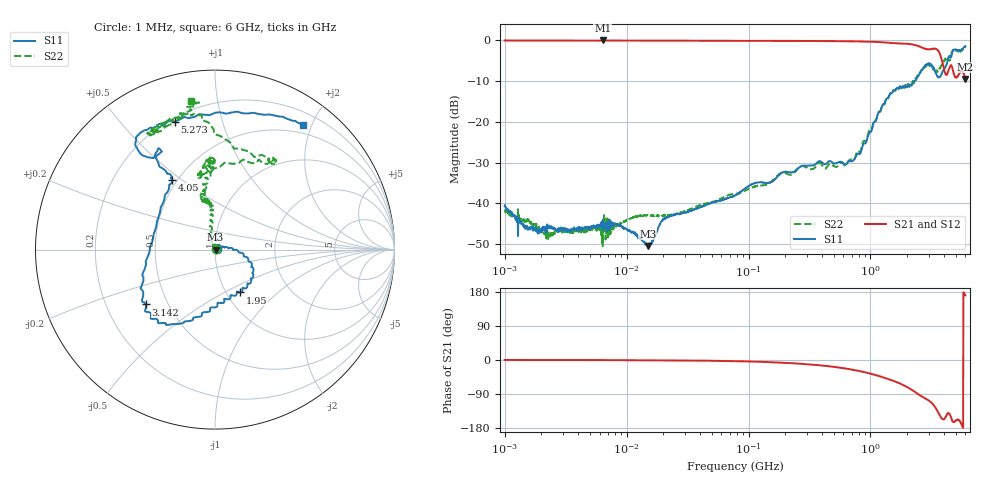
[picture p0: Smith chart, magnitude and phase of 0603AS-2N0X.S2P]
!s-Parameter Generated by FASTRON Sdn. Bhd.
!FASTRON P/N : 0603AS-2N0X
!Keysight Technologies: E5071C_MY46733604_B.14.02
!Date: Tue Nov 21 15:46:42 2023
!Version  :Rev01  Tue Nov 21 15:46:42 2023
!Data & Calibration Information:
!Freq  S11:SOLT2(ON)  S21:SOLT2(ON)  S12:SOLT2(ON)  S22:SOLT2(ON)
!PortZ  Port1:50+j0  Port2:50+j0
!When reading reference impedance value at option line is always used.
! Remarks : This data is being provided solely for informational purposes.
# Hz S dB R 50
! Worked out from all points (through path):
!   1601 points, 1 MHz to 6 GHz, reference 50 ohm
!   highest |S21| = -0.02 dB at 6.378 MHz (marker M1); lowest = -9.5 dB at 6 GHz (marker M2)
!   group delay of S21, straight-line fit = 94.1 ps
!   lowest |S11| = -50.5 dB at 14.93 MHz (marker M3), VSWR 1.01, Z = 50.3 + j7.26e-05 ohm
!   |S11| at or under -10 dB: start of sweep to 2.301 GHz
!   |S22| runs from -50.5 to -1.6 dB; largest |S21 - S12| = 0.0075
!   S11 on the Smith chart (normalised r, x): 1 MHz: 1.02, +0.01; 1.95 GHz: 1.16, -0.60; 3.142 GHz: 0.38, -0.30; 4.05 GHz: 0.47, +0.46; 5.273 GHz: 0.22, +0.71; 6 GHz: 0.37, +1.86
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1000000  -40.68 15.9  -0.04 0.1  -0.06 0.1  -41.49 20.4
1554926  -46.48 3.0  -0.04 -0.1  -0.06 0.0  -44.42 -8.8
2300516  -46.08 20.6  -0.05 -0.1  -0.06 -0.1  -47.76 27.9
4277066  -46.58 16.0  -0.06 -0.2  -0.06 -0.2  -46.72 19.0
6378092  -46.63 28.7  -0.02 -0.2  -0.07 -0.3  -50.51 -3.0
8700030  -45.31 19.6  -0.05 -0.4  -0.06 -0.4  -45.18 21.5
1.493236e7  -50.48 0.0  -0.05 -0.6  -0.06 -0.7  -42.86 15.6
1.823719e7  -45.87 21.3  -0.05 -0.8  -0.07 -0.7  -42.99 27.9
2.220078e7  -43.28 29.4  -0.06 -0.9  -0.07 -0.9  -42.85 36.4
7.757876e7  -38.08 48.4  -0.07 -3.0  -0.09 -3.0  -37.72 49.0
3.307917e8  -30.68 47.7  -0.15 -12.1  -0.16 -12.1  -31.63 77.3
7.246463e8  -29.41 26.7  -0.24 -26.0  -0.25 -26.1  -29.31 115.9
1.414819e9  -13.73 -19.2  -0.59 -51.0  -0.59 -51.0  -13.90 92.7
1.949935e9  -11.17 -59.8  -0.83 -69.5  -0.85 -69.5  -10.95 101.9
2.731395e9  -6.54 -117.9  -1.95 -98.9  -1.97 -98.8  -6.59 94.0
3.141603e9  -6.18 -141.5  -2.11 -111.6  -2.11 -111.6  -6.55 95.6
3.644712e9  -9.06 165.7  -2.81 -142.2  -2.81 -142.4  -7.29 96.0
4.049696e9  -6.82 121.5  -7.60 -155.0  -7.62 -155.1  -4.75 57.8
4.272437e9  -5.15 123.7  -8.15 -141.2  -8.16 -141.3  -4.51 59.4
4.824846e9  -2.30 124.3  -8.33 -163.6  -8.36 -163.7  -2.25 101.6
5.272524e9  -2.54 107.4  -8.39 -157.8  -8.42 -157.7  -2.75 119.0
6e9  -1.42 54.9  -9.45 170.5  -9.43 170.6  -1.55 99.0
